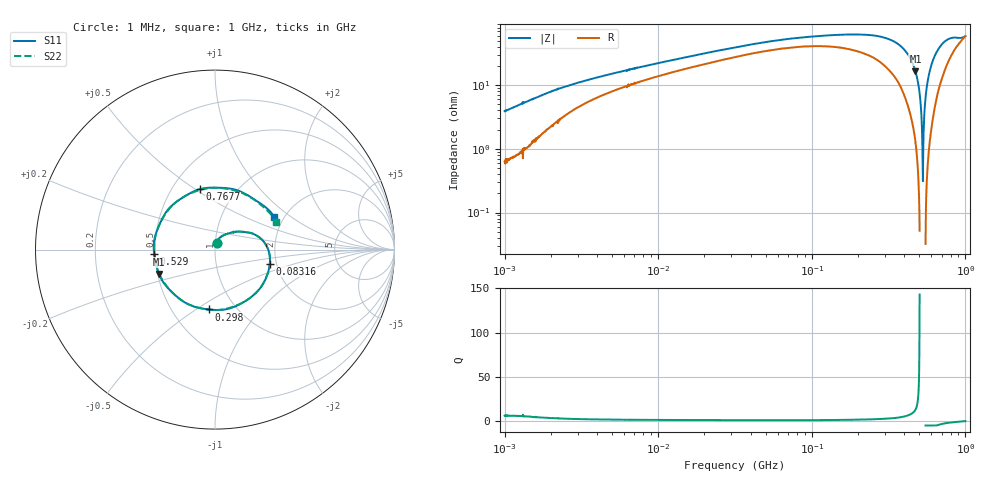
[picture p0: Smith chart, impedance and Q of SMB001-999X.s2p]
!s-Parameter Generated by FASTRON Sdn. Bhd.
!FASTRON P/N : SMB/001-999X
!Vector Network Analyser E5071C,MY46733604,B.14.02
!Date: Mon Jul 31 13:23:04 2023
!Data & Calibration Information:
!Freq	S11:SOLT2(ON)	S21:SOLT2(ON)	S12:SOLT2(ON)	S22:SOLT2(ON)
!PortZ  Port1:50+j0  Port2:50+j0
!When reading, reference impedance value at option line is always used.
! Remarks : This data is being provided solely for informational purposes.
# Hz S dB R 50
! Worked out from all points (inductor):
!   1601 points, 1 MHz to 1 GHz, reference 50 ohm
!   read as one part in series: L = 616 nH near 1.041 MHz
!   highest Q = 12.8 at 473 MHz (marker M1), where L = 5.52 nH
!   self-resonance near 528.4 MHz
!   S11 on the Smith chart (normalised r, x): 1 MHz: 1.01, +0.07; 83.16 MHz: 1.84, -0.32; 298 MHz: 0.75, -0.56; 529 MHz: 0.49, -0.03; 767.7 MHz: 0.68, +0.52; 1 GHz: 1.78, +0.75
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1000000  -28.66 76.4  -0.05 -2.3  -0.06 -2.4  -28.79 76.3
2163912  -22.34 65.9  -0.25 -4.8  -0.25 -4.8  -22.32 66.1
3167252  -20.08 56.8  -0.45 -6.2  -0.45 -6.1  -20.08 56.5
1.002882e7  -15.26 35.4  -1.20 -10.6  -1.20 -10.6  -15.20 35.3
3.163788e7  -11.74 14.7  -2.22 -19.1  -2.22 -19.0  -11.73 14.7
8.316394e7  -10.03 -14.3  -3.13 -34.7  -3.13 -34.7  -10.01 -14.7
1.00144e8  -9.86 -22.2  -3.25 -39.8  -3.25 -39.8  -9.85 -22.5
1.809276e8  -9.57 -54.2  -3.48 -65.3  -3.47 -65.3  -9.55 -54.9
2.42296e8  -9.42 -76.6  -3.54 -85.4  -3.54 -85.3  -9.50 -77.2
2.979702e8  -9.49 -96.2  -3.57 -104.0  -3.57 -104.0  -9.46 -97.2
3.171813e8  -9.47 -103.1  -3.58 -110.4  -3.58 -110.4  -9.46 -103.9
3.889559e8  -9.44 -127.8  -3.60 -134.6  -3.60 -134.6  -9.42 -129.1
4.729727e8  -9.35 -156.5  -3.62 -163.0  -3.62 -163.0  -9.39 -158.1
5.29014e8  -9.37 -176.1  -3.65 178.0  -3.65 178.0  -9.42 -177.3
5.821428e8  -9.33 166.6  -3.66 159.9  -3.66 159.9  -9.36 164.6
6.379281e8  -9.33 147.2  -3.69 140.9  -3.68 140.9  -9.37 145.6
7.123084e8  -9.34 122.5  -3.71 115.3  -3.71 115.4  -9.33 120.3
7.676511e8  -9.18 104.1  -3.74 96.4  -3.74 96.5  -9.28 101.9
8.192842e8  -9.23 86.8  -3.77 78.5  -3.78 78.6  -9.25 84.3
8.709173e8  -9.04 70.2  -3.83 60.7  -3.82 60.7  -9.15 67.5
9.409908e8  -8.89 47.2  -3.96 36.1  -3.96 36.1  -8.95 44.4
1e9  -8.50 28.9  -4.20 15.2  -4.19 15.3  -8.51 24.5
